(* Logix 5000 AddOnInstructionDefinition export YAI_Assy_151_120_EIP_Hz; software revision 21.03 *)

ADD_ON_INSTRUCTION YAI_Assy_151_120_EIP_Hz   (* revision 1.0, vendor Yaskawa America, Inc. *)
// YAI Assembly 151 and 120
// Help:
// This add-on instruction is for use with input assemblie 151 and output assemblies 120.
// Node_Input_Assy is defined as the node's input assembly integer array.
// Node_Output_Assy is defined as the node's output assembly integer array.
// Torque limit/reference, torque compensation and torque output variables are only available with A1000.
VAR_IN_OUT
   Node_Input_Assy : AB:ETHERNET_MODULE_INT_8Bytes:I:0; {required}   // Input assembly words
   Node_Output_Assy : AB:ETHERNET_MODULE_INT_24Bytes:O:0; {required}   // Output assembly words
END_VAR
VAR_INPUT
   RunFwd : BOOL; {visible}   // Forward run command
   RunRev : BOOL; {visible}   // Reverse run command
   MFI_3 : BOOL; {visible}   // Multi-function input 3
   MFI_4 : BOOL; {visible}   // Multi-function input 4
   MFI_5 : BOOL; {visible}   // Multi-function input 5
   MFI_6 : BOOL; {visible}   // Multi-function input 6
   MFI_7 : BOOL; {visible}   // Multi-function input 7
   MFI_8 : BOOL; {visible}   // Multi-function input 8
   External_Fault : BOOL;   // External fault command (EF0)
   FaultReset : BOOL; {visible}   // Fault reset command
   MFO_1 : BOOL; {visible}   // Multi-function output (M1-M2 for A/P1000, MA/MB/MC for V1000)
   MFO_2 : BOOL; {visible}   // Multi-function output (M3-M4 for A/P1000, P1 for V1000)
   MFO_3 : BOOL; {visible}   // Multi-function output (M5-M6 for A/P1000, P2 for V1000)
   Freq_Ref : REAL; {visible}   // Frequency reference command in Hz (xx.xx resolution)
   Digital_Output_Fault_Enable : BOOL;   // Bit to enable control of fault output relay over the network
END_VAR
VAR_OUTPUT
   Running : BOOL; {access Read Only, visible}   // Drive running forward status bit
   ZSP : BOOL; {access Read Only, visible}   // Drive zero speed status bit
   RunningRev : BOOL; {access Read Only, visible}   // Drive running reverse status bit
   Reset : BOOL; {access Read Only, visible}   // Drive reset command status bit
   At_Speed : BOOL; {access Read Only, visible}   // Drive at commanded speed status bit
   Ready : BOOL; {access Read Only, visible}   // Drive ready status bit
   Alarm : BOOL; {access Read Only, visible}   // Drive alarm status bit
   Faulted : BOOL; {access Read Only, visible}   // Drive faulted status bit
   UV : BOOL; {access Read Only}   // Drive in UV (undervoltage) state status bit
   MFO_1_Status : BOOL; {access Read Only, visible}   // Drive multi-function output 1 (M1-M2 for A/P1000, MA/MB/MC for V1000) status
   MFO_2_Status : BOOL; {access Read Only, visible}   // Drive multi-function output 1 (M3-M4 for A/P1000, P1 for V1000) status
   MFO_3_Status : BOOL; {access Read Only, visible}   // Drive multi-function output 1 (M5-M6 for A/P1000, P2 for V1000) status
   ZSV : BOOL; {access Read Only, visible}   // Drive zero servo completed status bit
   Motor_Speed : REAL; {access Read Only, visible}   // Motor speed in Hz (xx.xx resolution)
   Torque_Actual : REAL; {access Read Only, visible}   // Drive torque output in % (xxx.x resolution)
   Output_Freq : REAL; {access Read Only, visible}   // Drive output frequency in Hz (xx.xx resolution)
   Output_Current : REAL; {access Read Only, visible}   // Drive output current in A (xxx.x resolution)
   RUN_Alarm : BOOL; {access Read Only}   // Motor 2 run command issued while running alarm
END_VAR
VAR_INPUT
   Custom_Out_1 : INT;
   Custom_Out_2 : INT;
   Custom_Out_3 : INT;
   Custom_Out_4 : INT;
   Custom_Out_5 : INT;
   Custom_Out_6 : INT;
   Custom_Out_7 : INT;
   Custom_Out_8 : INT;
   Custom_Out_9 : INT;
   Custom_Out_10 : INT;
END_VAR
VAR_OUTPUT
   OPE : BOOL; {access Read Only}   // OPE alarm/fault present
   NetCtrlStatus : BOOL; {access Read Only, visible}   // Drive network run source status bit (1 = source coming from network)
END_VAR
VAR
   FRef_Convert : DINT;
   FOut_Convert : REAL;
   FOut_Temp : REAL;
   TRef_Convert : INT;
   TComp_Convert : INT;
   TOut_Convert : REAL;
   TOut_Temp : REAL;
   IOut_Temp : REAL;
   IOut_Convert : REAL;
   AO1_Convert : INT;
   AO2_Convert : INT;
   Motor_Speed_Temp : REAL;
   Motor_Speed_Convert : REAL;
   Freq_Cmd_Temp : REAL;
   Freq_Cmd_Convert : REAL;
   AI1_Temp : REAL;
   AI1_Convert : REAL;
   AI2_Temp : REAL; {access None}
   AI2_Convert : REAL; {access None}
   AI3_Temp : REAL; {access None}
   AI3_Convert : REAL; {access None}
END_VAR

ROUTINE Logic   (* ladder *)
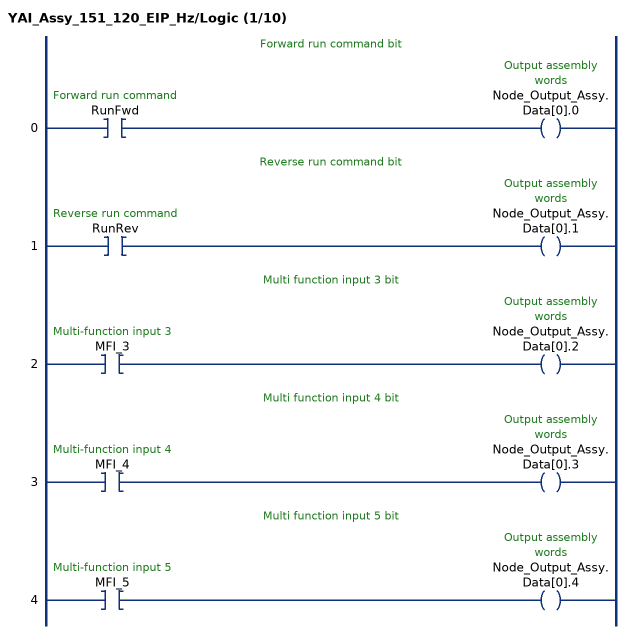
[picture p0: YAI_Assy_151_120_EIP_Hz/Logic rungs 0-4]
   // Forward run command bit
   0: XIC(RunFwd)OTE(Node_Output_Assy.Data[0].0);
   // Reverse run command bit
   1: XIC(RunRev)OTE(Node_Output_Assy.Data[0].1);
   // Multi function input 3 bit
   2: XIC(MFI_3)OTE(Node_Output_Assy.Data[0].2);
   // Multi function input 4 bit
   3: XIC(MFI_4)OTE(Node_Output_Assy.Data[0].3);
   // Multi function input 5 bit
   4: XIC(MFI_5)OTE(Node_Output_Assy.Data[0].4);
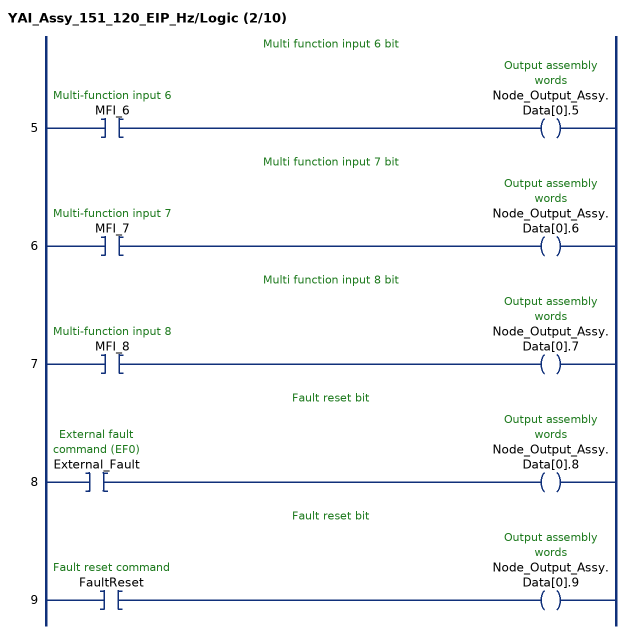
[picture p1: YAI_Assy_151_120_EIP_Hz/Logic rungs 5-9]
   // Multi function input 6 bit
   5: XIC(MFI_6)OTE(Node_Output_Assy.Data[0].5);
   // Multi function input 7 bit
   6: XIC(MFI_7)OTE(Node_Output_Assy.Data[0].6);
   // Multi function input 8 bit
   7: XIC(MFI_8)OTE(Node_Output_Assy.Data[0].7);
   // Fault reset bit
   8: XIC(External_Fault)OTE(Node_Output_Assy.Data[0].8);
   // Fault reset bit
   9: XIC(FaultReset)OTE(Node_Output_Assy.Data[0].9);
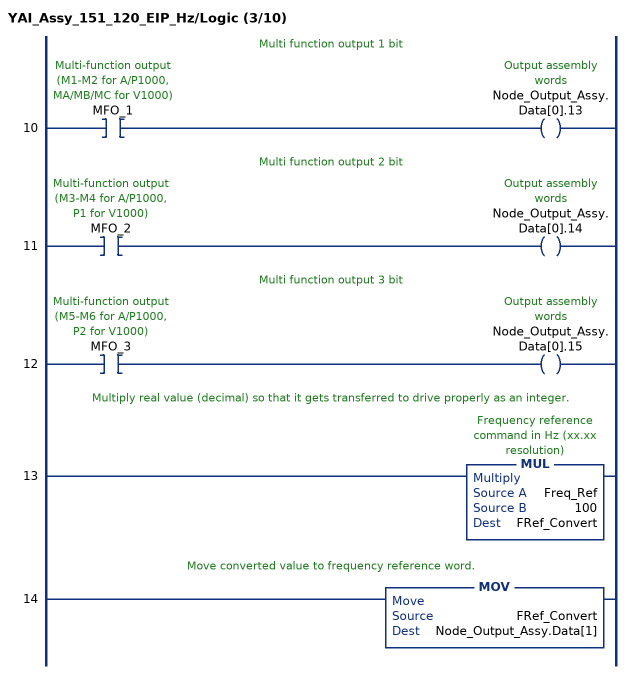
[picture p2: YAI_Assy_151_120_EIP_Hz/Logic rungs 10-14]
   // Multi function output 1 bit
   10: XIC(MFO_1)OTE(Node_Output_Assy.Data[0].13);
   // Multi function output 2 bit
   11: XIC(MFO_2)OTE(Node_Output_Assy.Data[0].14);
   // Multi function output 3 bit
   12: XIC(MFO_3)OTE(Node_Output_Assy.Data[0].15);
   // Multiply real value (decimal) so that it gets transferred to drive properly as an integer.
   13: MUL(Freq_Ref,100,FRef_Convert);
   // Move converted value to frequency reference word.
   14: MOV(FRef_Convert,Node_Output_Assy.Data[1]);
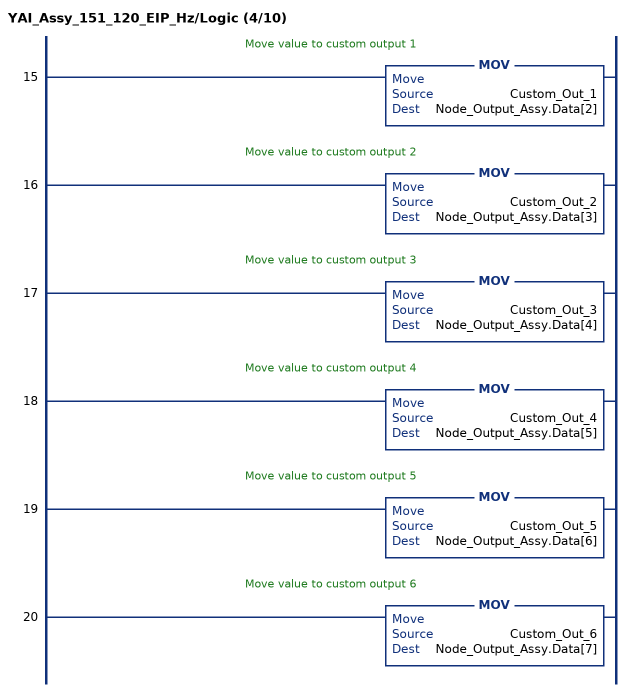
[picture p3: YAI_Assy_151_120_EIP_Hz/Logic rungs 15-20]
   // Move value to custom output 1
   15: MOV(Custom_Out_1,Node_Output_Assy.Data[2]);
   // Move value to custom output 2
   16: MOV(Custom_Out_2,Node_Output_Assy.Data[3]);
   // Move value to custom output 3
   17: MOV(Custom_Out_3,Node_Output_Assy.Data[4]);
   // Move value to custom output 4
   18: MOV(Custom_Out_4,Node_Output_Assy.Data[5]);
   // Move value to custom output 5
   19: MOV(Custom_Out_5,Node_Output_Assy.Data[6]);
   // Move value to custom output 6
   20: MOV(Custom_Out_6,Node_Output_Assy.Data[7]);
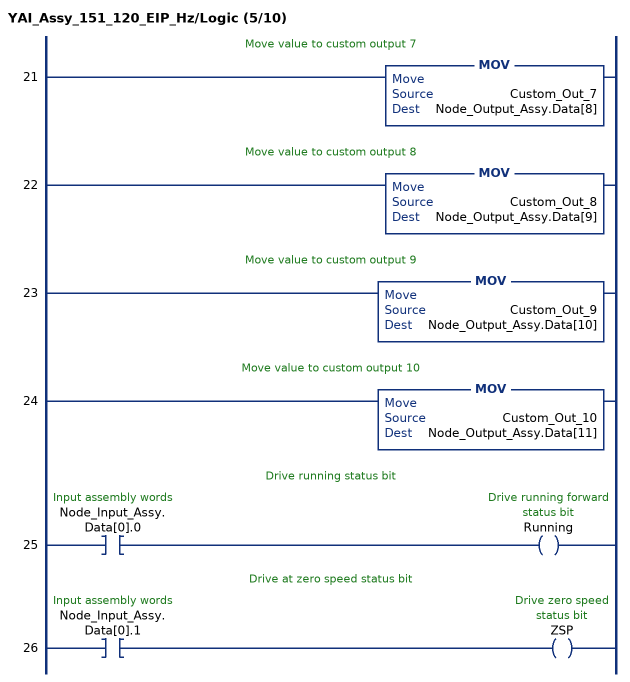
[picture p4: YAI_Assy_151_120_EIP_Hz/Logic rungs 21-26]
   // Move value to custom output 7
   21: MOV(Custom_Out_7,Node_Output_Assy.Data[8]);
   // Move value to custom output 8
   22: MOV(Custom_Out_8,Node_Output_Assy.Data[9]);
   // Move value to custom output 9
   23: MOV(Custom_Out_9,Node_Output_Assy.Data[10]);
   // Move value to custom output 10
   24: MOV(Custom_Out_10,Node_Output_Assy.Data[11]);
   // Drive running status bit
   25: XIC(Node_Input_Assy.Data[0].0)OTE(Running);
   // Drive at zero speed status bit
   26: XIC(Node_Input_Assy.Data[0].1)OTE(ZSP);
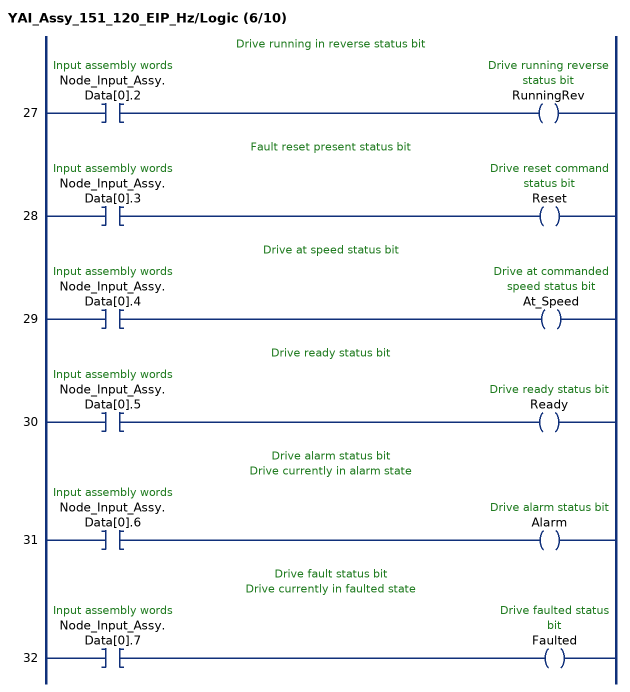
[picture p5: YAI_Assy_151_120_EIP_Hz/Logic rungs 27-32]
   // Drive running in reverse status bit
   27: XIC(Node_Input_Assy.Data[0].2)OTE(RunningRev);
   // Fault reset present status bit
   28: XIC(Node_Input_Assy.Data[0].3)OTE(Reset);
   // Drive at speed status bit
   29: XIC(Node_Input_Assy.Data[0].4)OTE(At_Speed);
   // Drive ready status bit
   30: XIC(Node_Input_Assy.Data[0].5)OTE(Ready);
   // Drive alarm status bit
   // Drive currently in alarm state
   31: XIC(Node_Input_Assy.Data[0].6)OTE(Alarm);
   // Drive fault status bit
   // Drive currently in faulted state
   32: XIC(Node_Input_Assy.Data[0].7)OTE(Faulted);
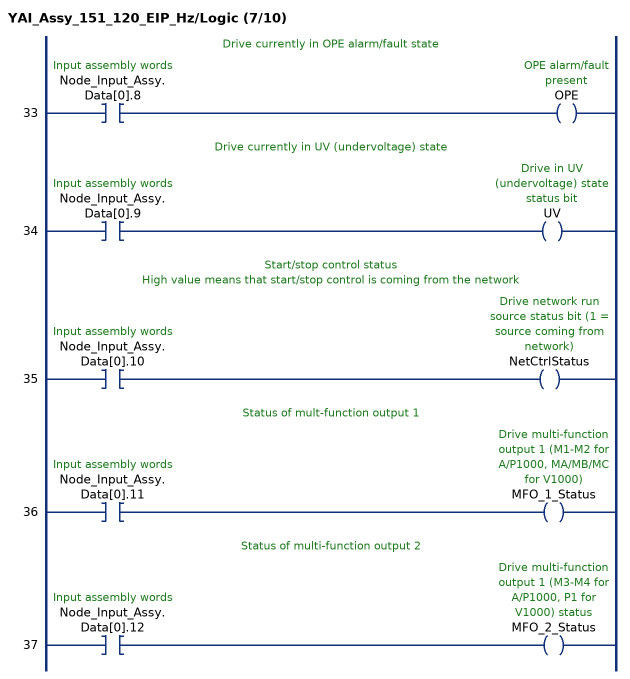
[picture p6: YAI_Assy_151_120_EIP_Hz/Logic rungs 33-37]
   // Drive currently in OPE alarm/fault state
   33: XIC(Node_Input_Assy.Data[0].8)OTE(OPE);
   // Drive currently in UV (undervoltage) state
   34: XIC(Node_Input_Assy.Data[0].9)OTE(UV);
   // Start/stop control status
   // High value means that start/stop control is coming from the network
   35: XIC(Node_Input_Assy.Data[0].10)OTE(NetCtrlStatus);
   // Status of mult-function output 1
   36: XIC(Node_Input_Assy.Data[0].11)OTE(MFO_1_Status);
   // Status of multi-function output 2
   37: XIC(Node_Input_Assy.Data[0].12)OTE(MFO_2_Status);
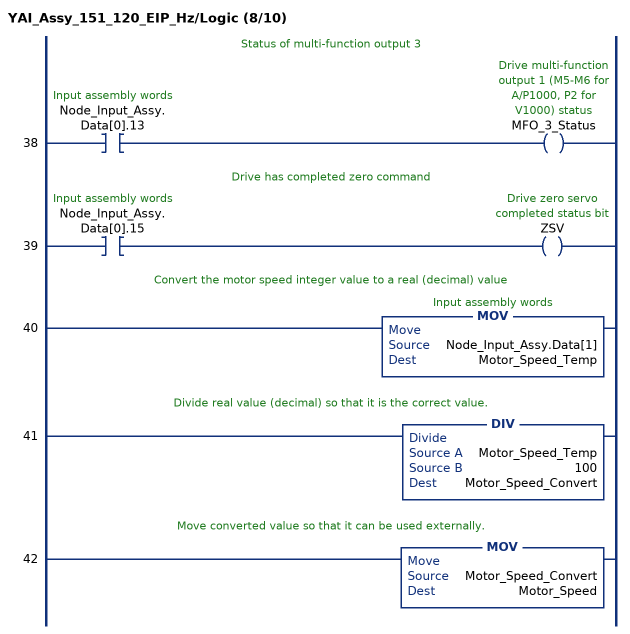
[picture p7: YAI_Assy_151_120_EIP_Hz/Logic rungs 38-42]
   // Status of multi-function output 3
   38: XIC(Node_Input_Assy.Data[0].13)OTE(MFO_3_Status);
   // Drive has completed zero command
   39: XIC(Node_Input_Assy.Data[0].15)OTE(ZSV);
   // Convert the motor speed integer value to a real (decimal) value
   40: MOV(Node_Input_Assy.Data[1],Motor_Speed_Temp);
   // Divide real value (decimal) so that it is the correct value.
   41: DIV(Motor_Speed_Temp,100,Motor_Speed_Convert);
   // Move converted value so that it can be used externally.
   42: MOV(Motor_Speed_Convert,Motor_Speed);
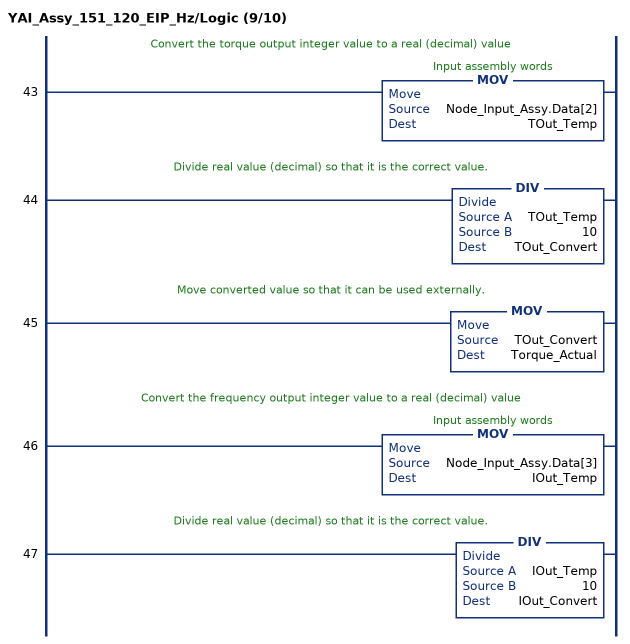
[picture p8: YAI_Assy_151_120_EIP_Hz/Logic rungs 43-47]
   // Convert the torque output integer value to a real (decimal) value
   43: MOV(Node_Input_Assy.Data[2],TOut_Temp);
   // Divide real value (decimal) so that it is the correct value.
   44: DIV(TOut_Temp,10,TOut_Convert);
   // Move converted value so that it can be used externally.
   45: MOV(TOut_Convert,Torque_Actual);
   // Convert the frequency output integer value to a real (decimal) value
   46: MOV(Node_Input_Assy.Data[3],IOut_Temp);
   // Divide real value (decimal) so that it is the correct value.
   47: DIV(IOut_Temp,10,IOut_Convert);
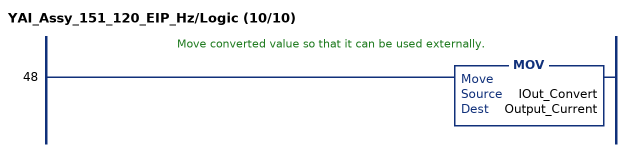
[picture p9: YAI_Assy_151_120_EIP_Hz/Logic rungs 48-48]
   // Move converted value so that it can be used externally.
   48: MOV(IOut_Convert,Output_Current);
END_ROUTINE
END_ADD_ON_INSTRUCTION
